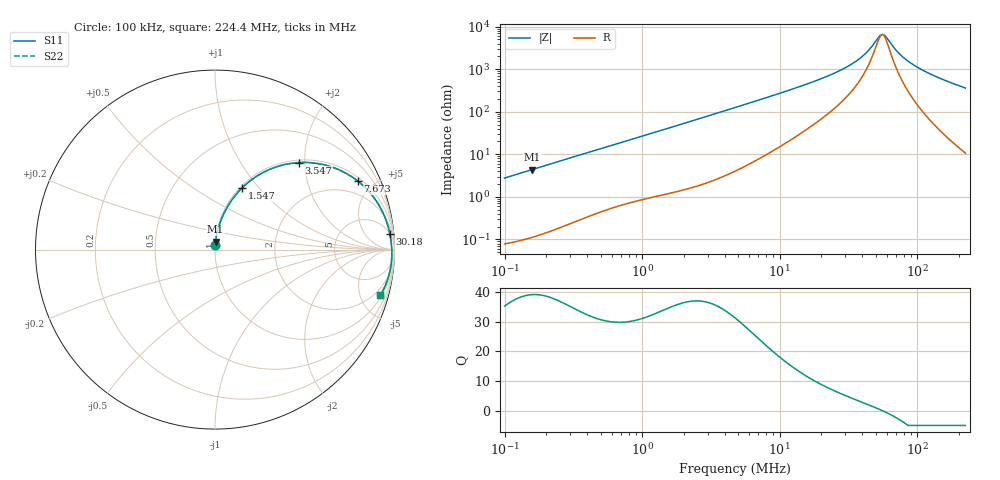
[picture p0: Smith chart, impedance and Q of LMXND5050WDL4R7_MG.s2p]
! LMXND5050WDL4R7_MG  S-PARAMETER MODEL  ( General Type )
! Model Generated by TAIYO YUDEN Corporation (https://www.yuden.co.jp/en/)
! Version 1.0
! TAIYO YUDEN Control No. 191023NI43SB-FBB
! Copyright(c) 2019 TAIYO YUDEN CO.,LTD. All Rights Reserved.
! Product Description (link to TY-COMPAS)
! https://ds.yuden.co.jp/TYCOMPAS/or/detail?pn=LMXND5050WDL4R7MMG&u=M
! Products Name : Inductors
! Characteristics :
!  Inductance : 4.7 uH , SRF(min) : 37 MHz , DC Resistance(max) : 0.066 Ohm
!  Rated Current : Saturation :2700 mA , Temp Rise : 2000 mA (40 degC)
!  Case Size : 4.9 x 4.9 / 0.193 x 0.193 [mm/inch] , Thickness : 2.4 / 0.094 [mm/inch]
!  (Conditions: Temperature = 25 degC , DC Bias Current/Voltage = 0A / 0V)
! External Node Assignments :
!  1  o---GGG---o  2
! GND o---------o GND
! Frequency Range : 0.1MHz  -  224.402193MHz  [ 402 STEP ]
# MHz S RI R 50
! Freq[MHz].  S11 Real  S11 Imag  S21 Real  S21 Imag  S12 Real  S12 Imag  S22 Real  S22 Imag
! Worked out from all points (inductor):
!   401 points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, 100 kHz to 224.4 MHz, reference 50 ohm
!   read as one part in series: L = 4.39 uH near 103.9 kHz
!   highest Q = 39.1 at 158.9 kHz (marker M1), where L = 4.39 uH
!   self-resonance near 54.89 MHz
!   S11 on the Smith chart (normalised r, x): 100 kHz: 1.00, +0.06; 1.547 MHz: 1.02, +0.82; 3.547 MHz: 1.05, +1.87; 7.673 MHz: 1.18, +4.09; 30.18 MHz: 5, +21; 224.4 MHz: 1.21, -7.19
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0.1  0.00154 0.0275  0.9985 -0.0275  0.9985 -0.0275  0.00154 0.0275
0.158877  0.00303 0.0436  0.997 -0.0436  0.997 -0.0436  0.00303 0.0436
0.364164  0.0127 0.0979  0.9873 -0.0979  0.9873 -0.0979  0.0127 0.0979
0.77272  0.0472 0.1959  0.9528 -0.1959  0.9528 -0.1959  0.0472 0.1959
1.326154  0.1171 0.3068  0.8829 -0.3068  0.8829 -0.3068  0.1171 0.3068
1.547443  0.1504 0.3433  0.8496 -0.3433  0.8496 -0.3433  0.1504 0.3433
2.275967  0.2699 0.4305  0.7301 -0.4305  0.7301 -0.4305  0.2699 0.4305
3.546909  0.4668 0.4849  0.5332 -0.4849  0.5332 -0.4849  0.4668 0.4849
4.737111  0.6065 0.4728  0.3935 -0.4728  0.3935 -0.4728  0.6065 0.4728
7.67278  0.7968 0.3809  0.2032 -0.3809  0.2032 -0.3809  0.7968 0.3809
11.06946  0.8865 0.2883  0.1135 -0.2883  0.1135 -0.2883  0.8865 0.2883
17.25085  0.9445 0.1861  0.0555 -0.1861  0.0555 -0.1861  0.9445 0.1861
30.18284  0.9747 0.0865  0.0253 -0.0865  0.0253 -0.0865  0.9747 0.0865
35.90527  0.9792 0.0607  0.0208 -0.0607  0.0208 -0.0607  0.9792 0.0607
41.09615  0.9817 0.0417  0.0183 -0.0417  0.0183 -0.0417  0.9817 0.0417
54.88639  0.9848 0.00217  0.0152 -0.00217  0.0152 -0.00217  0.9848 0.00217
58.15638  0.9851 -0.00573  0.0149 0.00573  0.0149 0.00573  0.9851 -0.00573
62.8214  0.9853 -0.0164  0.0147 0.0164  0.0147 0.0164  0.9853 -0.0164
76.18743  0.9847 -0.0438  0.0153 0.0438  0.0153 0.0438  0.9847 -0.0438
97.90203  0.9813 -0.0826  0.0187 0.0826  0.0187 0.0826  0.9813 -0.0826
141.2425  0.9672 -0.1491  0.0328 0.1491  0.0328 0.1491  0.9672 -0.1491
224.4022  0.9219 -0.254  0.0781 0.254  0.0781 0.254  0.9219 -0.254
